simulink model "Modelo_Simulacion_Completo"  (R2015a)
settings: Solver=ode45  StartTime=0  StopTime=.1  FixedStep=Ts  MaxStep=1e-6  RelTol=1e-6  AbsTol=1e-6
PreLoadFcn:
  | assignin('base','Ts',[5e-6])
undefined symbols (not defined in the file): A, axis, behind, by, degrees, established, Flux, Ion, linkage, Lithium, magnets, modified, Park, phase, Ts, V
libraries: simulink x7, powerlib x7, dspsigops x3, electricdrivelib x1, powerlib_meascontrol x1

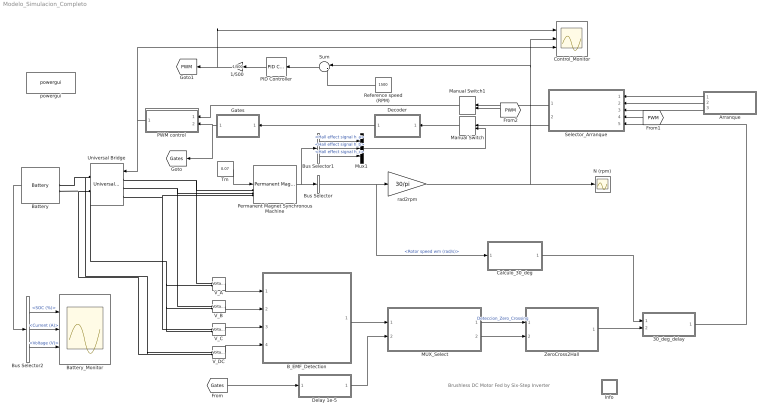
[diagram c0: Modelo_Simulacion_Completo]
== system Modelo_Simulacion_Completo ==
  note: Brushless DC Motor Fed by Six-Step Inverter
  " MUX_Select" : Subsystem
  "1/500 " : Gain  Gain=1/500
  30_deg_delay : Subsystem
  Arranque : Subsystem
  B_EMF_Detection : Subsystem
  Battery : electricdrivelib/Extra Sources/Battery  BatType=Lithium-Ion  ShowDetailedParameters=off  NomV=24  NomQ=6.5  SOC=100  PresetModel=on  MaxQ=6.5  FullV=27.9357  Dis_rate=2.8261  R=0.036923  Normal_OP=5.8783  expZone="[25.9293     0.319348]"  current=[6.5 13 32.5]  Units=Time  Batt_Tr=30
  Battery_Monitor : Scope  NumInputPorts=3
  Bus Selector : BusSelector  OutputSignals=Rotor speed wm (rad/s)
  Bus Selector1 : BusSelector  OutputSignals=Hall effect signal h_a,Hall effect signal h_b,Hall effect signal h_c
  Bus Selector2 : BusSelector  OutputSignals=SOC (%),Current (A),Voltage (V)
  Calculo_30_deg : Subsystem
  Control_Monitor : Scope  NumInputPorts=3
  Decoder : Subsystem
  Delay 1e-5 : Subsystem
  Gates : Subsystem
  Info : Subsystem
  Manual Switch : ManualSwitch
  Manual Switch1 : ManualSwitch
  Mux1 : Mux  Inputs=3
  N (rpm) : Scope
  PID Controller : simulink/Continuous/PID Controller  Controller=PID  TimeDomain=Continuous-time  SampleTime=-1  IntegratorMethod=Forward Euler  FilterMethod=Forward Euler  Form=Parallel  UseFilter=on  ControllerParametersSource=internal  P=500  I=0.1  D=0.08  N=1  InitialConditionSource=internal  InitialConditionForIntegrator=0  InitialConditionForFilter=0  ExternalReset=none  LimitOutput=off  UpperSaturationLimit=inf  LowerSaturationLimit=-inf  LinearizeAsGain=on  AntiWindupMode=none  Kb=1  TrackingMode=off  Kt=1  PParamMin=[]  PParamMax=[]  IParamMin=[]  IParamMax=[]  DParamMin=[]  DParamMax=[]  NParamMin=[]  NParamMax=[]  KbParamMin=[]  KbParamMax=[]  KtParamMin=[]  KtParamMax=[]  POutMin=[]  POutMax=[]  IOutMin=[]  IOutMax=[]  DOutMin=[]  DOutMax=[]  NOutMin=[]  NOutMax=[]  KbOutMin=[]  KbOutMax=[]  KtOutMin=[]  KtOutMax=[]  IntegratorOutMin=[]  IntegratorOutMax=[]  FilterOutMin=[]  FilterOutMax=[]  SumOutMin=[]  SumOutMax=[]  SumI1OutMin=[]  SumI1OutMax=[]  SumI2OutMin=[]  SumI2OutMax=[]  SumI3OutMin=[]  SumI3OutMax=[]  SumDOutMin=[]  SumDOutMax=[]  SaturationOutMin=[]  SaturationOutMax=[]  IntegratorContinuousStateAttributes=''  IntegratorStateMustResolveToSignalObject=off  IntegratorRTWStateStorageClass=Auto  FilterContinuousStateAttributes=''  FilterStateMustResolveToSignalObject=off  FilterRTWStateStorageClass=Auto  DifferentiatorICPrevScaledInput=0  DifferentiatorOutMin=[]  DifferentiatorOutMax=[]
  PWM control : Subsystem
  Permanent Magnet Synchronous Machine : powerlib/Machines/Permanent Magnet Synchronous Machine  NbPhases=3  FluxDistribution=Trapezoidal  RotorType=Round  MechanicalLoad=Torque Tm  PresetModel=No  ShowDetailedParameters=on  MeasurementBus=off  Resistance=2.015  Inductance=0.0023  dqInductances=[8.5e-3, 8.5e-3]  La=0.000835  MachineConstant=Flux linkage established by magnets (V.s)  Flux=0.0115228  VoltageCst=7.24  TorqueCst=0.069137  Flat=120  Mechanical=[4.43465e-06 0.000303448 3]  PolePairs=4  InitialConditions=[0,0, 0,0]  InitialConditions5ph=[0 0 0 0 0 0]  TsPowergui=0  TsBlock=-1  RefAngle=90 degrees behind phase A axis (modified Park)
  Reference speed (RPM) : Constant  Value=1500
  Selector_Arranque : Subsystem
  Sum : Sum  Inputs=|-+
  Tm : Constant  Value=0.07
  Universal Bridge : powerlib/Power Electronics/Universal Bridge  Arms=3  SnubberResistance=5000  SnubberCapacitance=1e-6  Device=MOSFET / Diodes  Ron=1e-3  Lon=0  ForwardVoltages="[  0  0  ]"  ForwardVoltage=0  GTOparameters=[ 10e-6 , 20e-6 ]  IGBTparameters=[ 1e-6 , 2e-6 ]  Measurements=None  Measurements_2=None  converterType=Rectifier
  V_A : powerlib/Measurements/Voltage Measurement  PhasorSimulation=off  OutputType=Complex  PSBequivalent=0
  V_B : powerlib/Measurements/Voltage Measurement  PhasorSimulation=off  OutputType=Complex  PSBequivalent=0
  V_C : powerlib/Measurements/Voltage Measurement  PhasorSimulation=off  OutputType=Complex  PSBequivalent=0
  V_DC : powerlib/Measurements/Voltage Measurement  PhasorSimulation=off  OutputType=Complex  PSBequivalent=0
  ZeroCross2Hall : Subsystem
  powergui : powerlib/powergui  Priority=2  SimulationMode=Discrete  SolverType=Tustin/Backward Euler (TBE)  SampleTime=Ts  frequency=60  SPID=off  DisableSnubberDevices=off  DisableRonSwitches=off  DisableVfSwitches=off  SwTol=0  DisplayEquations=off  Interpol=off  methode=off  Ts=0  FunctionMessages=off  echomessages=off  HookPort=off  EnableUseOfTLC=off  x0status=blocks  frequencyindice=0  Pbase=100e6  ErrMax=1e-4  Iterations=50  UnitsV=kV  UnitsW=MW  buscounter=0  RestoreLinks=warning  ResistiveCurrentMeasurement=off  Frange=[0:2:500]  Ylog=off  Xlog=on  ShowGrid=off  save=off  variable=ZData  structure=0  ZoomFFT=on  StartTime=0.0  cycles=1  DisplayStyle=1  fundamental=60  FreqAxis=off  MaxFrequency=1000  frequencyindicesteady=1  RmsSteady=1  display=off
  rad2rpm : Gain  Gain=30/pi
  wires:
  Tm/1 -> Permanent Magnet Synchronous Machine/1
  Decoder/1(emf_abc) -> Gates/1("emf_abc ")
  rad2rpm/1 -> Control_Monitor/2, Sum/1, N (rpm)/1
  Permanent Magnet Synchronous Machine/1 -> Bus Selector1/1, Bus Selector/1
  Battery/1 -> Bus Selector2/1
  Bus Selector2/1 -> Battery_Monitor/1  "<SOC (%)>"
  Bus Selector2/2 -> Battery_Monitor/2  "<Current (A)>"
  Bus Selector2/3 -> Battery_Monitor/3  "<Voltage (V)>"
  Reference speed (RPM)/1 -> Sum/2
  Sum/1 -> PID Controller/1
  PID Controller/1 -> "1/500 "/1
  "1/500 "/1 -> Control_Monitor/1, [PWM]
  Gates/1(Gates) -> [Gates], PWM control/2(Gates)
  PWM control/1(Pulsos) -> Control_Monitor/3, Universal Bridge/1
  Bus Selector/1 -> Calculo_30_deg/1(N_rad_s), rad2rpm/1  "<Rotor speed wm (rad/s)>"
  Bus Selector1/1 -> Mux1/1  "<Hall effect signal h_a>"
  Bus Selector1/2 -> Mux1/2  "<Hall effect signal h_b>"
  Bus Selector1/3 -> Mux1/3  "<Hall effect signal h_c>"
  [Gates] -> Delay 1e-5/1(Gates)
  B_EMF_Detection/1(B_EMF) -> " MUX_Select"/1(bEMF_detect)
  Delay 1e-5/1(Gates_delay) -> " MUX_Select"/2(Gates)
  " MUX_Select"/1(Zero_Crossing) -> ZeroCross2Hall/1(zero_crossing)  "Deteccion_Zero_Crossing"
  Calculo_30_deg/1(Delay) -> 30_deg_delay/1(30_deg)
  " MUX_Select"/2(Trigger) -> ZeroCross2Hall/2(trigger)
  Arranque/1(Trigger) -> Selector_Arranque/1(Trigger)
  Manual Switch/1 -> Decoder/1("Hall ")
  Mux1/1 -> Manual Switch/2
  V_A/1 -> B_EMF_Detection/1(V_A)
  V_B/1 -> B_EMF_Detection/2(V_B)
  V_C/1 -> B_EMF_Detection/3(V_C)
  V_DC/1 -> B_EMF_Detection/4(V_DC)
  ZeroCross2Hall/1(Hall) -> 30_deg_delay/2(Hall)
  Arranque/2(PWM_Arranque) -> Selector_Arranque/2(PWM_Arranque)
  Arranque/3(Hall_Arranque) -> Selector_Arranque/3(Hal_Arranque)
  30_deg_delay/1(Hall_Delay) -> Selector_Arranque/5(Hall_Regulacion)
  Selector_Arranque/2(Hall) -> Manual Switch/1
  [PWM] -> Selector_Arranque/4(PWM_Regulacion)
  Manual Switch1/1 -> PWM control/1(V control)
  Selector_Arranque/1(PWM) -> Manual Switch1/1
  [PWM] -> Manual Switch1/2
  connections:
  Universal Bridge/LConn1 -- V_A/LConn1 -- Permanent Magnet Synchronous Machine/LConn1
  Universal Bridge/LConn2 -- Permanent Magnet Synchronous Machine/LConn2 -- V_B/LConn1
  Universal Bridge/LConn3 -- V_C/LConn1 -- Permanent Magnet Synchronous Machine/LConn3
  Universal Bridge/RConn1 -- V_DC/LConn1 -- Battery/LConn1
  Universal Bridge/RConn2 -- V_C/LConn2 -- V_B/LConn2 -- V_A/LConn2 -- V_DC/LConn2 -- Battery/LConn2

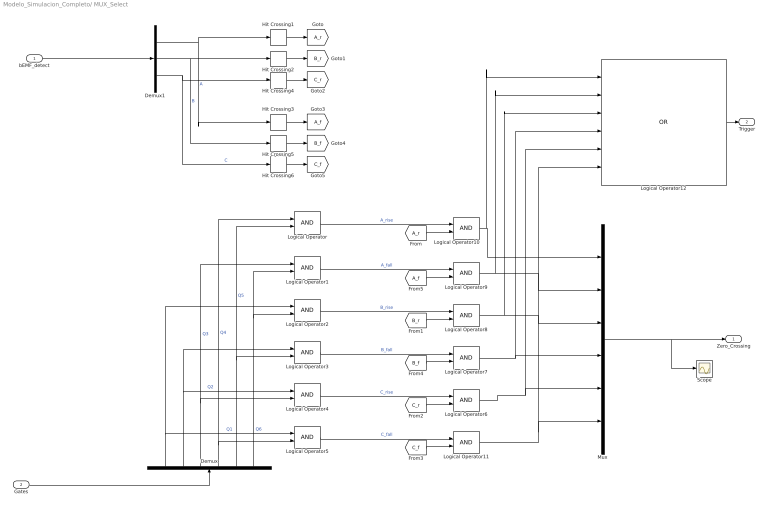
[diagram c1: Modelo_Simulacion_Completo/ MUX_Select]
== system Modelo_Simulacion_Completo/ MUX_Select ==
  bEMF_detect : Inport
  Gates : Inport  Port=2
  Demux : Demux  Outputs=6
  Demux1 : Demux  Outputs=3
  Hit Crossing1 : HitCross  HitCrossingDirection=rising
  Hit Crossing2 : HitCross  HitCrossingDirection=rising
  Hit Crossing3 : HitCross  HitCrossingDirection=falling
  Hit Crossing4 : HitCross  HitCrossingDirection=rising
  Hit Crossing5 : HitCross  HitCrossingDirection=falling
  Hit Crossing6 : HitCross  HitCrossingDirection=falling
  Logical Operator{,1..11} (12 alike) : Logic  IconShape=distinctive  AllPortsSameDT=off  OutDataTypeStr=boolean
  Logical Operator12 : Logic  Operator=OR  Inputs=6  AllPortsSameDT=off  OutDataTypeStr=boolean
  Mux : Mux  Inputs=6
  Scope : Scope
  Zero_Crossing : Outport
  Trigger : Outport  Port=2
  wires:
  Gates/1 -> Demux/1
  Demux/1 -> Logical Operator5/1, Logical Operator2/1  "Q1"
  Demux/2 -> Logical Operator4/1, Logical Operator3/1  "Q2"
  Demux/3 -> Logical Operator4/2, Logical Operator1/1  "Q3"
  Demux/4 -> Logical Operator5/2, Logical Operator/1  "Q4"
  Demux/5 -> Logical Operator3/2, Logical Operator/2  "Q5"
  Demux/6 -> Logical Operator2/2, Logical Operator1/2  "Q6"
  Logical Operator2/1 -> Logical Operator8/1  "B_rise"
  Logical Operator3/1 -> Logical Operator7/1  "B_fall"
  Logical Operator/1 -> Logical Operator10/1  "A_rise"
  Logical Operator1/1 -> Logical Operator9/1  "A_fall"
  Logical Operator4/1 -> Logical Operator6/1  "C_rise"
  Logical Operator5/1 -> Logical Operator11/1  "C_fall"
  bEMF_detect/1 -> Demux1/1
  Demux1/1 -> Hit Crossing3/1, Hit Crossing1/1  "A"
  Demux1/2 -> Hit Crossing5/1, Hit Crossing2/1  "B"
  Demux1/3 -> Hit Crossing6/1, Hit Crossing4/1  "C"
  Hit Crossing1/1 -> [A_r]
  Hit Crossing2/1 -> [B_r]
  Hit Crossing4/1 -> [C_r]
  Hit Crossing3/1 -> [A_f]
  Hit Crossing5/1 -> [B_f]
  Hit Crossing6/1 -> [C_f]
  [A_r] -> Logical Operator10/2
  [A_f] -> Logical Operator9/2
  [B_r] -> Logical Operator8/2
  [B_f] -> Logical Operator7/2
  [C_r] -> Logical Operator6/2
  [C_f] -> Logical Operator11/2
  Mux/1 -> Scope/1, Zero_Crossing/1
  Logical Operator6/1 -> Logical Operator12/5, Mux/5
  Logical Operator11/1 -> Mux/6, Logical Operator12/6
  Logical Operator7/1 -> Logical Operator12/4, Mux/4
  Logical Operator8/1 -> Logical Operator12/3, Mux/3
  Logical Operator9/1 -> Logical Operator12/2, Mux/2
  Logical Operator10/1 -> Logical Operator12/1, Mux/1
  Logical Operator12/1 -> Trigger/1

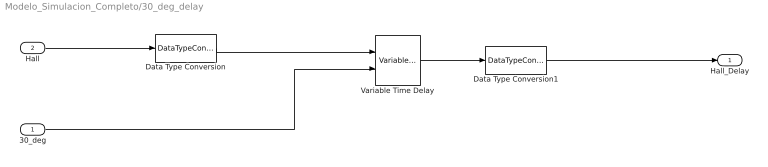
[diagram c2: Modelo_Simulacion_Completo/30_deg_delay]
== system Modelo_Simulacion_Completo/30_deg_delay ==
  30_deg : Inport
  Hall : Inport  Port=2
  Data Type Conversion : DataTypeConversion  OutDataTypeStr=double
  Data Type Conversion1 : DataTypeConversion  OutDataTypeStr=boolean
  Variable Time Delay : VariableTransportDelay  MaximumDelay=10
  Hall_Delay : Outport
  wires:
  Hall/1 -> Data Type Conversion/1
  Data Type Conversion/1 -> Variable Time Delay/1
  30_deg/1 -> Variable Time Delay/2
  Variable Time Delay/1 -> Data Type Conversion1/1
  Data Type Conversion1/1 -> Hall_Delay/1

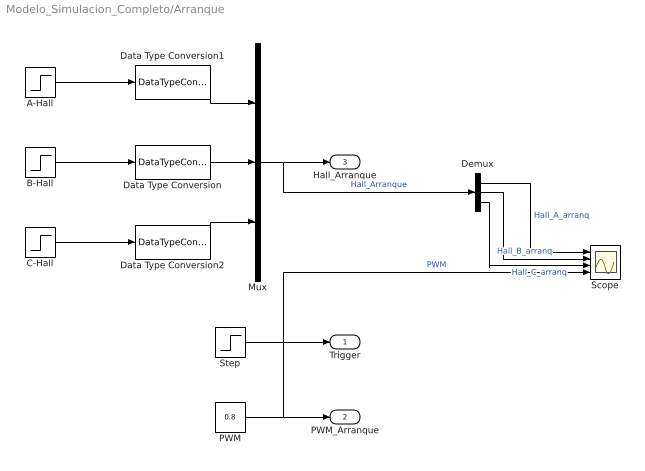
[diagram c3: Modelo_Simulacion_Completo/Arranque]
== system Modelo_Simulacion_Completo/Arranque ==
  A-Hall : Step  Time=8.364E-3  Before=1  After=0  SampleTime=0
  B-Hall : Step  Time=5.8145E-3  SampleTime=0
  C-Hall : Step  Time=10.8E-3  SampleTime=0
  Data Type Conversion : DataTypeConversion  OutDataTypeStr=boolean
  Data Type Conversion1 : DataTypeConversion  OutDataTypeStr=boolean
  Data Type Conversion2 : DataTypeConversion  OutDataTypeStr=boolean
  Demux : Demux  Outputs=3
  Mux : Mux  Inputs=3
  PWM : Constant  Value=0.8
  Scope : Scope  NumInputPorts=4
  Step : Step  Time=13.25E-3  Before=0.5  After=-0.5  SampleTime=0
  Trigger : Outport
  PWM_Arranque : Outport  Port=2
  Hall_Arranque : Outport  Port=3
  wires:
  B-Hall/1 -> Data Type Conversion/1
  C-Hall/1 -> Data Type Conversion2/1
  A-Hall/1 -> Data Type Conversion1/1
  Data Type Conversion/1 -> Mux/2
  Data Type Conversion1/1 -> Mux/1
  Data Type Conversion2/1 -> Mux/3
  Mux/1 -> Demux/1, Hall_Arranque/1  "Hall_Arranque"
  Step/1 -> Trigger/1
  PWM/1 -> Scope/4, PWM_Arranque/1  "PWM"
  Demux/1 -> Scope/1  "Hall_A_arranq"
  Demux/2 -> Scope/2  "Hall_B_arranq"
  Demux/3 -> Scope/3  "Hall_C_arranq"

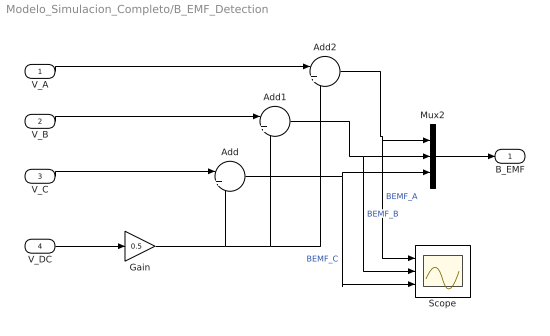
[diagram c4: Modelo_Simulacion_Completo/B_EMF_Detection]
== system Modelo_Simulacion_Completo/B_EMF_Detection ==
  V_A : Inport
  V_B : Inport  Port=2
  V_C : Inport  Port=3
  V_DC : Inport  Port=4
  Add : Sum  Inputs=|+-
  Add1 : Sum  Inputs=|+-
  Add2 : Sum  Inputs=|+-
  Gain : Gain  Gain=0.5
  Mux2 : Mux  Inputs=3
  Scope : Scope  NumInputPorts=3
  B_EMF : Outport
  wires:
  V_DC/1 -> Gain/1
  V_A/1 -> Add2/1
  V_B/1 -> Add1/1
  V_C/1 -> Add/1
  Gain/1 -> Add2/2, Add1/2, Add/2
  Mux2/1 -> B_EMF/1
  Add2/1 -> Scope/1, Mux2/1  "BEMF_A"
  Add1/1 -> Scope/2, Mux2/2  "BEMF_B"
  Add/1 -> Scope/3, Mux2/3  "BEMF_C"

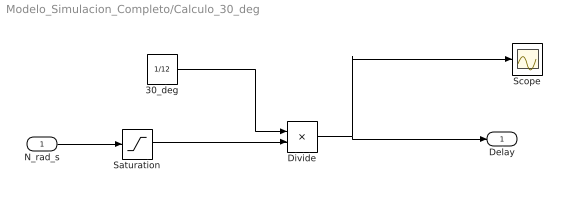
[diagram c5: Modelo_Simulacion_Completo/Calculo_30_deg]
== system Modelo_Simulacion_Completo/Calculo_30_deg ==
  N_rad_s : Inport
  30_deg : Constant  Value=1/12
  Divide : Product  Inputs=*/
  Saturation : Saturate  UpperLimit=inf  LowerLimit=10
  Scope : Scope
  Delay : Outport
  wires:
  30_deg/1 -> Divide/1
  Divide/1 -> Scope/1, Delay/1
  N_rad_s/1 -> Saturation/1
  Saturation/1 -> Divide/2

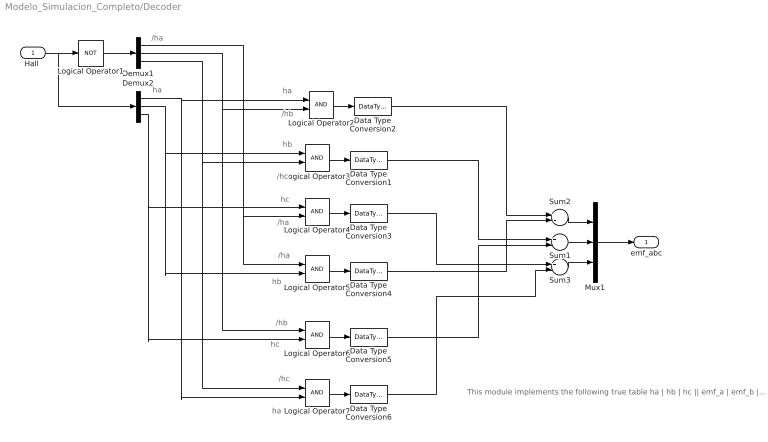
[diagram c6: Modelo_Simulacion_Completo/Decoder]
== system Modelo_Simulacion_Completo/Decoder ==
  note: /ha
  note: ha
  note: ha
  note: /hb
  note: hb
  note: /hc
  note: hc
  note: /ha
  note: /ha
  note: hb
  note: /hb
  note: hc
  note: /hc
  note: ha
  note: This module implements the following true table ha | hb | hc || emf_a | emf_b | emf_c -------------------------------------------------------------------------------- 0 0 0 0 0 0 0 0 1 0 -1 +1 0 1 0 -1 +1 0 0 1 1 -1 0 +1 1 0 0 +1 0 -1 1 0 1 +1 -1 0 1 1 0 0 +1 -1 1 1 1 0 0 0
  "Hall " : Inport
  Data Type Conversion{1..6} (6 alike) : DataTypeConversion
  Demux1 : Demux  Outputs=3
  Demux2 : Demux  Outputs=3
  Logical Operator1 : Logic  Operator=NOT  AllPortsSameDT=off  OutDataTypeStr=boolean
  Logical Operator{2..7} (6 alike) : Logic  AllPortsSameDT=off  OutDataTypeStr=boolean
  Mux1 : Mux  Inputs=3
  Sum1 : Sum  Inputs=+-  OutDataTypeStr=double
  Sum2 : Sum  Inputs=+-  OutDataTypeStr=double
  Sum3 : Sum  Inputs=+-  OutDataTypeStr=double
  emf_abc : Outport
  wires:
  "Hall "/1 -> Logical Operator1/1, Demux2/1
  Logical Operator1/1 -> Demux1/1
  Demux2/3 -> Logical Operator4/1, Logical Operator6/2
  Demux2/2 -> Logical Operator3/1, Logical Operator5/2
  Demux2/1 -> Logical Operator2/1, Logical Operator7/2
  Demux1/3 -> Logical Operator3/2, Logical Operator7/1
  Demux1/2 -> Logical Operator2/2, Logical Operator6/1
  Demux1/1 -> Logical Operator4/2, Logical Operator5/1
  Logical Operator2/1 -> Data Type Conversion2/1
  Sum2/1 -> Mux1/1
  Sum1/1 -> Mux1/2
  Sum3/1 -> Mux1/3
  Mux1/1 -> emf_abc/1
  Logical Operator3/1 -> Data Type Conversion1/1
  Logical Operator4/1 -> Data Type Conversion3/1
  Logical Operator5/1 -> Data Type Conversion4/1
  Logical Operator6/1 -> Data Type Conversion5/1
  Logical Operator7/1 -> Data Type Conversion6/1
  Data Type Conversion2/1 -> Sum2/1
  Data Type Conversion4/1 -> Sum2/2
  Data Type Conversion1/1 -> Sum1/1
  Data Type Conversion5/1 -> Sum1/2
  Data Type Conversion3/1 -> Sum3/1
  Data Type Conversion6/1 -> Sum3/2

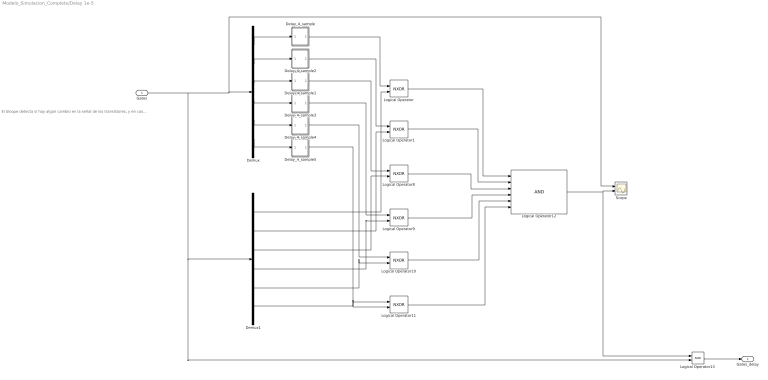
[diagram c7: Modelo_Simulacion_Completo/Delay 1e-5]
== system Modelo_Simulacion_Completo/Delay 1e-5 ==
  note: El bloque detecta si hay algún cambio en la señal de los transistores, y en caso afirmativo (momento de conmutación), coloca todas las señales a cero durante 1e-5 segundos para que no exista error en la detección de cruce por cero.
  Gates : Inport
  Delay_4_sample : Subsystem
  Delay_4_sample1 : Subsystem
  Delay_4_sample2 : Subsystem
  Delay_4_sample3 : Subsystem
  Delay_4_sample4 : Subsystem
  Delay_4_sample5 : Subsystem
  Demux : Demux  Outputs=6
  Demux1 : Demux  Outputs=6
  Logical Operator{,1,8..11} (6 alike) : Logic  Operator=NXOR  IconShape=distinctive  AllPortsSameDT=off  OutDataTypeStr=boolean
  Logical Operator12 : Logic  Inputs=6  IconShape=distinctive  AllPortsSameDT=off  OutDataTypeStr=boolean
  Logical Operator13 : Logic  AllPortsSameDT=off  OutDataTypeStr=boolean
  Scope : Scope  NumInputPorts=2
  Gates_delay : Outport
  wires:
  Demux/3 -> Delay_4_sample1/1(In)
  Demux/2 -> Delay_4_sample2/1(In)
  Gates/1 -> Demux1/1, Logical Operator13/2, Scope/1, Demux/1
  Demux1/5 -> Logical Operator10/2
  Demux1/6 -> Logical Operator11/2
  Demux1/4 -> Logical Operator9/2
  Demux1/3 -> Logical Operator8/2
  Demux1/2 -> Logical Operator1/2
  Demux1/1 -> Logical Operator/2
  Logical Operator8/1 -> Logical Operator12/3
  Logical Operator/1 -> Logical Operator12/1
  Logical Operator1/1 -> Logical Operator12/2
  Logical Operator9/1 -> Logical Operator12/4
  Logical Operator10/1 -> Logical Operator12/5
  Logical Operator11/1 -> Logical Operator12/6
  Logical Operator12/1 -> Logical Operator13/1, Scope/2
  Logical Operator13/1 -> Gates_delay/1
  Delay_4_sample2/1(Out) -> Logical Operator1/1
  Delay_4_sample1/1(Out) -> Logical Operator8/1
  Demux/1 -> Delay_4_sample/1(In)
  Delay_4_sample/1(Out) -> Logical Operator/1
  Demux/4 -> Delay_4_sample3/1(In)
  Delay_4_sample3/1(Out) -> Logical Operator9/1
  Delay_4_sample4/1(Out) -> Logical Operator10/1
  Delay_4_sample5/1(Out) -> Logical Operator11/1
  Demux/6 -> Delay_4_sample5/1(In)
  Demux/5 -> Delay_4_sample4/1(In)

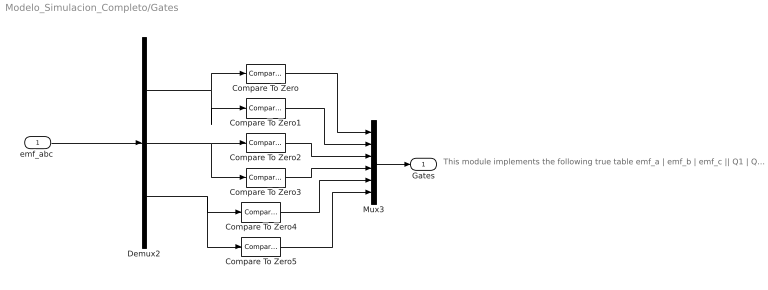
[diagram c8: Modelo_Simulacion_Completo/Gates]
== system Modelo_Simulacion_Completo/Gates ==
  note: This module implements the following true table emf_a | emf_b | emf_c || Q1 | Q2 | Q3 | Q4 | Q5 | Q6 ------------------------------------------------------------------------------------------------------------------ 0 0 0 0 0 0 0 0 0 0 -1 +1 0 0 0 1 1 0 -1 +1 0 0 1 1 0 0 0 -1 0 +1 0 1 0 0 1 0 +1 0 -1 1 0 0 0 0 1 +1 -1 0 1 0 0 1 0 0 0 +1 -1 0 0 1 0 0 1 0 0 0 0 0 0 0 0 0
  "emf_abc " : Inport
  Compare To Zero : simulink/Logic and Bit Operations/Compare To Zero  relop=>  OutDataTypeStr=boolean  ZeroCross=off
  Compare To Zero1 : simulink/Logic and Bit Operations/Compare To Zero  relop=<  OutDataTypeStr=boolean  ZeroCross=off
  Compare To Zero2 : simulink/Logic and Bit Operations/Compare To Zero  relop=>  OutDataTypeStr=boolean  ZeroCross=off
  Compare To Zero3 : simulink/Logic and Bit Operations/Compare To Zero  relop=<  OutDataTypeStr=boolean  ZeroCross=off
  Compare To Zero4 : simulink/Logic and Bit Operations/Compare To Zero  relop=>  OutDataTypeStr=boolean  ZeroCross=off
  Compare To Zero5 : simulink/Logic and Bit Operations/Compare To Zero  relop=<  OutDataTypeStr=boolean  ZeroCross=off
  Demux2 : Demux  Outputs=3
  Mux3 : Mux  Inputs=6
  Gates : Outport
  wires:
  "emf_abc "/1 -> Demux2/1
  Mux3/1 -> Gates/1
  Demux2/1 -> Compare To Zero/1, Compare To Zero1/1
  Demux2/2 -> Compare To Zero2/1, Compare To Zero3/1
  Demux2/3 -> Compare To Zero4/1, Compare To Zero5/1
  Compare To Zero/1 -> Mux3/1
  Compare To Zero1/1 -> Mux3/2
  Compare To Zero2/1 -> Mux3/3
  Compare To Zero3/1 -> Mux3/4
  Compare To Zero4/1 -> Mux3/5
  Compare To Zero5/1 -> Mux3/6

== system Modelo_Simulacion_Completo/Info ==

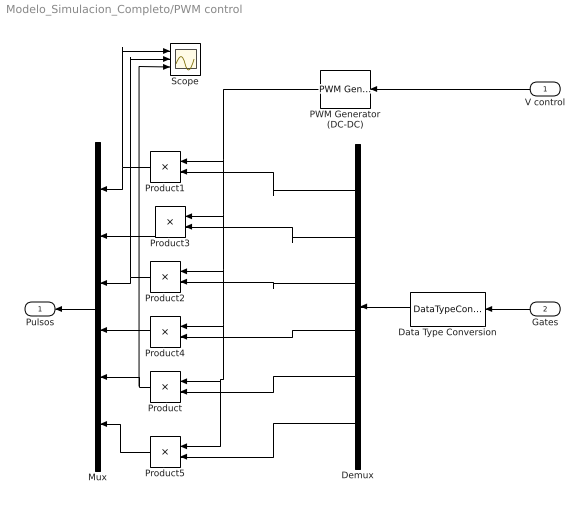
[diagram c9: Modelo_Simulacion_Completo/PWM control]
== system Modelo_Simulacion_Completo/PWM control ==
  V control : Inport
  Gates : Inport  Port=2
  Data Type Conversion : DataTypeConversion  OutDataTypeStr=double
  Demux : Demux  Outputs=6
  Mux : Mux  Inputs=6
  PWM Generator (DC-DC) : powerlib_meascontrol/Pulse & Signal Generators/PWM Generator (DC-DC)  Fsw=50000  Ts=0
  Product{,1..5} (6 alike) : Product
  Scope : Scope  NumInputPorts=3
  Pulsos : Outport
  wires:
  Gates/1 -> Data Type Conversion/1
  Data Type Conversion/1 -> Demux/1
  Mux/1 -> Pulsos/1
  Product1/1 -> Scope/1, Mux/1
  Product2/1 -> Scope/2, Mux/3
  Product/1 -> Scope/3, Mux/5
  Demux/5 -> Product/2
  Demux/3 -> Product2/2
  Demux/1 -> Product1/2
  V control/1 -> PWM Generator (DC-DC)/1
  PWM Generator (DC-DC)/1 -> Product3/1, Product4/1, Product5/1, Product/1, Product2/1, Product1/1
  Product5/1 -> Mux/6
  Demux/6 -> Product5/2
  Product4/1 -> Mux/4
  Demux/4 -> Product4/2
  Product3/1 -> Mux/2
  Demux/2 -> Product3/2

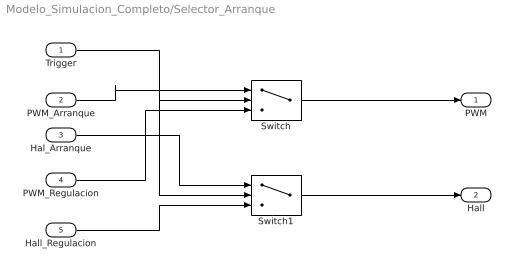
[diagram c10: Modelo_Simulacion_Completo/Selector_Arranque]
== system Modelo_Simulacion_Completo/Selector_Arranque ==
  Trigger : Inport
  PWM_Arranque : Inport  Port=2
  Hal_Arranque : Inport  Port=3
  PWM_Regulacion : Inport  Port=4
  Hall_Regulacion : Inport  Port=5
  Switch : Switch  Criteria=u2 > Threshold
  Switch1 : Switch  Criteria=u2 > Threshold
  PWM : Outport
  Hall : Outport  Port=2
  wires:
  Trigger/1 -> Switch1/2, Switch/2
  Hall_Regulacion/1 -> Switch1/3
  PWM_Regulacion/1 -> Switch/3
  Hal_Arranque/1 -> Switch1/1
  PWM_Arranque/1 -> Switch/1
  Switch/1 -> PWM/1
  Switch1/1 -> Hall/1

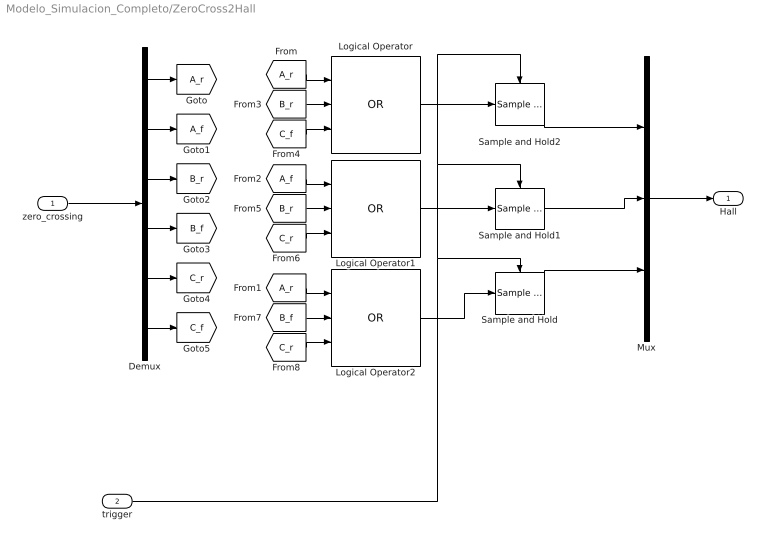
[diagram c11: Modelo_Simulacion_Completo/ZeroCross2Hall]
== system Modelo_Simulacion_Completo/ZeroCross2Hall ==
  zero_crossing : Inport
  trigger : Inport  Port=2
  Demux : Demux  Outputs=6
  Logical Operator : Logic  Operator=OR  Inputs=3  IconShape=distinctive  AllPortsSameDT=off  OutDataTypeStr=boolean
  Logical Operator1 : Logic  Operator=OR  Inputs=3  IconShape=distinctive  AllPortsSameDT=off  OutDataTypeStr=boolean
  Logical Operator2 : Logic  Operator=OR  Inputs=3  IconShape=distinctive  AllPortsSameDT=off  OutDataTypeStr=boolean
  Mux : Mux  Inputs=3
  Sample and Hold : dspsigops/Sample and Hold  trig=Rising edge  initCond=0  latchinput=off
  Sample and Hold1 : dspsigops/Sample and Hold  trig=Rising edge  initCond=0  latchinput=off
  Sample and Hold2 : dspsigops/Sample and Hold  trig=Rising edge  initCond=0  latchinput=off
  Hall : Outport
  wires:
  zero_crossing/1 -> Demux/1
  Mux/1 -> Hall/1
  trigger/1 -> Sample and Hold/Trigger, Sample and Hold1/Trigger, Sample and Hold2/Trigger
  Logical Operator2/1 -> Sample and Hold/1
  Sample and Hold/1 -> Mux/3
  Sample and Hold1/1 -> Mux/2
  Sample and Hold2/1 -> Mux/1
  Logical Operator1/1 -> Sample and Hold1/1
  Logical Operator/1 -> Sample and Hold2/1
  Demux/1 -> [A_r]
  Demux/6 -> [C_f]
  Demux/3 -> [B_r]
  Demux/2 -> [A_f]
  Demux/4 -> [B_f]
  Demux/5 -> [C_r]
  [A_r] -> Logical Operator2/1
  [A_r] -> Logical Operator/1
  [A_f] -> Logical Operator1/1
  [B_r] -> Logical Operator/2
  [C_f] -> Logical Operator/3
  [B_r] -> Logical Operator1/2
  [C_r] -> Logical Operator1/3
  [C_r] -> Logical Operator2/3
  [B_f] -> Logical Operator2/2

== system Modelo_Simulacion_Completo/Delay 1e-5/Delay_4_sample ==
  In : Inport
  Memory{2..3,14,22} (4 alike) : Memory
  Out : Outport
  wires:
  Memory3/1 -> Memory14/1
  Memory2/1 -> Memory3/1
  Memory22/1 -> Memory2/1
  In/1 -> Memory22/1
  Memory14/1 -> Out/1

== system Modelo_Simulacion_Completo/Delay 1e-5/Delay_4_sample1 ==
  In : Inport
  Memory{2..3,14,22} (4 alike) : Memory
  Out : Outport
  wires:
  Memory3/1 -> Memory14/1
  Memory2/1 -> Memory3/1
  Memory22/1 -> Memory2/1
  In/1 -> Memory22/1
  Memory14/1 -> Out/1

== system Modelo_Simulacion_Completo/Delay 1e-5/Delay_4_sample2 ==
  In : Inport
  Memory{2..3,14,22} (4 alike) : Memory
  Out : Outport
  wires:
  Memory3/1 -> Memory14/1
  Memory2/1 -> Memory3/1
  Memory22/1 -> Memory2/1
  In/1 -> Memory22/1
  Memory14/1 -> Out/1

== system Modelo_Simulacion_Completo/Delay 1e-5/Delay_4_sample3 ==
  In : Inport
  Memory{2..3,14,22} (4 alike) : Memory
  Out : Outport
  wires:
  Memory3/1 -> Memory14/1
  Memory2/1 -> Memory3/1
  Memory22/1 -> Memory2/1
  In/1 -> Memory22/1
  Memory14/1 -> Out/1

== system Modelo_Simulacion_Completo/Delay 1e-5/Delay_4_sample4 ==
  In : Inport
  Memory{2..3,14,22} (4 alike) : Memory
  Out : Outport
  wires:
  Memory3/1 -> Memory14/1
  Memory2/1 -> Memory3/1
  Memory22/1 -> Memory2/1
  In/1 -> Memory22/1
  Memory14/1 -> Out/1

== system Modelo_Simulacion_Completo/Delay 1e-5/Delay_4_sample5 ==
  In : Inport
  Memory{2..3,14,22} (4 alike) : Memory
  Out : Outport
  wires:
  Memory3/1 -> Memory14/1
  Memory2/1 -> Memory3/1
  Memory22/1 -> Memory2/1
  In/1 -> Memory22/1
  Memory14/1 -> Out/1
